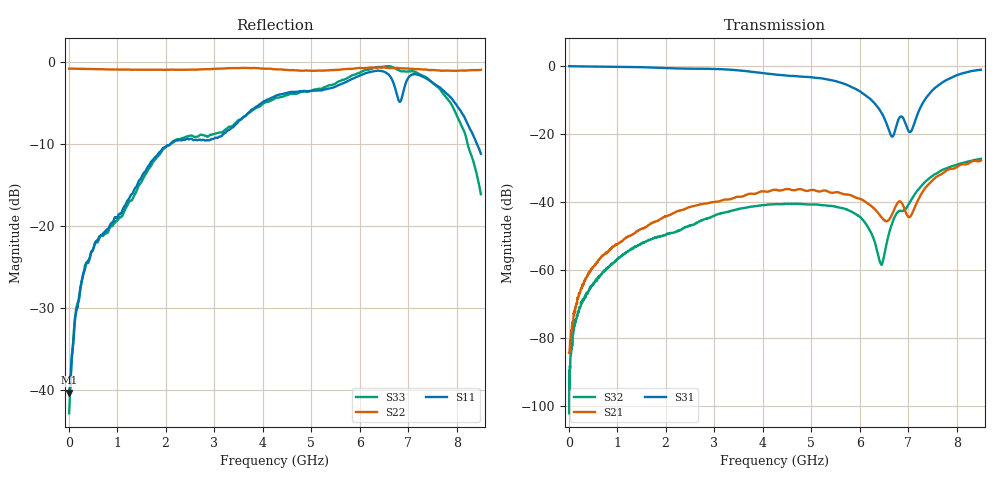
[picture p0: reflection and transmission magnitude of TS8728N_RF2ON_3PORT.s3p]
!Created with skrf (http://scikit-rf.org).
# GHz S RI R 50.0
!freq ReS11 ImS11 ReS12 ImS12 ReS13 ImS13
! ReS21 ImS21 ReS22 ImS22 ReS23 ImS23
! ReS31 ImS31 ReS32 ImS32 ReS33 ImS33
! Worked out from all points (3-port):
!   1601 points, 10 MHz to 8.5 GHz, reference 50 ohm
!   strongest paths, dB at 10 MHz, 2.132 GHz, 4.255 GHz, 6.378 GHz, 8.5 GHz:
!     S31: -0.1, -0.7, -2.5, -12.2, -1.1
!     S21: -84.3, -43.5, -36.4, -43.1, -27.8
!     S32: -102.0, -49.1, -40.6, -55.2, -27.3
!   lowest |S11| = -40.3 dB at 10 MHz (marker M1), VSWR 1.02, Z = 51 - j0.177 ohm
!   |S11| at or under -10 dB: start of sweep to 2.089 GHz; 8.422 GHz to end of sweep
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0.01  0.00952 -0.00174  -2.72e-05 4.02e-05  0.9878 -0.00539
      2.22e-05 5.68e-05  -0.9158 0.00477  1.54e-05 4.22e-06
      0.9877 -0.00553  -1.87e-06 -7.68e-06  0.0071 -0.00136
0.3124562  -0.00418 -0.0524  -3.75e-05 0.000649  0.9726 -0.1097
           -5.41e-05 0.000636  -0.9091 0.0897  -0.000136 -0.000322
           0.9726 -0.1097  -0.00014 -0.00034  -0.0028 -0.0524
0.9385938  -0.0314 -0.1062  -0.000447 0.00222  0.9182 -0.3133
           -0.000449 0.00222  -0.8578 0.293  -0.0012 -0.000527
           0.9179 -0.3131  -0.00117 -0.000562  -0.0355 -0.0987
4.255  -0.6133 -0.1092  0.00556 0.0141  0.0353 -0.7451
       0.00562 0.0141  -0.2504 0.8735  0.00127 0.00918
       0.0337 -0.7452  0.00131 0.00921  -0.5987 0.077
5.852181  -0.646 0.4617  0.0103 0.00677  -0.323 -0.3559
          0.0103 0.00676  0.248 0.88  0.00601 0.0038
          -0.3226 -0.3558  0.00601 0.00379  -0.4867 0.6806
6.446481  -0.503 0.731  0.00437 0.00408  -0.1684 -0.1212
          0.00439 0.00414  0.3694 0.8498  0.000135 0.00124
          -0.1679 -0.1212  0.000175 0.00119  -0.2405 0.907
6.722406  -0.2427 0.6704  -0.000167 0.00805  0.0137 -0.1056
          -0.000183 0.00807  0.4451 0.8118  -0.00445 0.00407
          0.0137 -0.106  -0.00443 0.00406  -0.0518 0.9219
7.046087  -0.3761 0.7415  -0.00119 0.00602  0.0491 -0.0947
          -0.00119 0.006  0.5207 0.7519  -0.00763 0.00679
          0.0494 -0.0947  -0.0076 0.00683  0.1858 0.8618
7.597937  0.2263 0.6855  -0.00808 0.0223  0.3513 -0.3558
          -0.0081 0.0223  0.6025 0.661  -0.00742 0.0255
          0.3527 -0.3552  -0.00741 0.0255  0.5799 0.4158
8.5  0.1394 0.2394  0.0136 0.0384  -0.0493 -0.8744
     0.0136 0.0384  0.7688 0.4691  0.0279 0.033
     -0.0489 -0.8749  0.0279 0.033  0.1428 -0.0651
